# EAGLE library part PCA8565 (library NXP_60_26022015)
Real time clock/calendar The PCA8565 is a CMOS real time clock and calendar optimized for low power consumption. A programmable clock output, interrupt output and voltage-low detector are also provided. All address and data are transferred serially via a two-line bidirectional I2C-bus. Maximum bus speed is 400 kbit/s. The built-in word address register is incremented automatically after each written or read data byte. AEC-Q100 compliant (PCA8565TS) for automotive applications. AAL Eindhoven MK
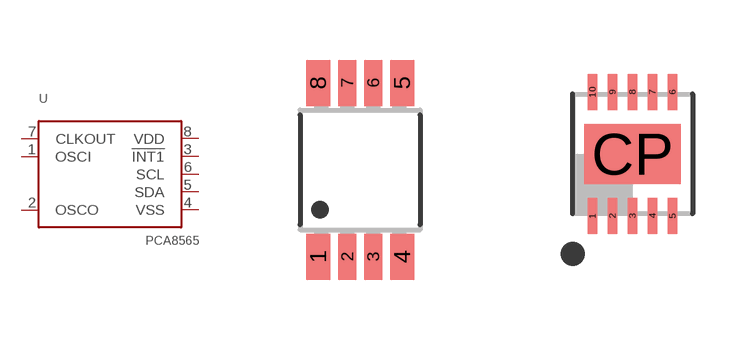
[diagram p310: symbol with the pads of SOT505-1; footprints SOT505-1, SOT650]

Designator prefix U

## PCA8565TS  [SOT505-1]
1  OSCI  pas
2  OSCO  pas
3  !INT1!  out
4  VSS  pwr
5  SDA
6  SCL  in
7  CLKOUT  pwr
8  VDD  pwr

## PCA8565BS  [SOT650]
1  OSCI  pas
2  OSCO  pas
4  !INT1!  out
5  VSS  pwr
6  SDA
7  SCL  in
8  CLKOUT  pwr
9  VDD  pwr

## Footprint SOT505-1 (pad centres in mm)
SOT505-1 TSSOP8: plastic thin shrink small outline package; 8 leads; body width 3 mm JEDEC: -- IEC: --
smd 0.6 x 1.15: 1 -1.05,-2.175; 4 1.05,-2.175; 5 1.05,2.175; 8 -1.05,2.175
smd 0.45 x 1.15: 2 -0.325,-2.175; 3 0.325,-2.175; 6 0.325,2.175; 7 -0.325,2.175

## Footprint SOT650 (pad centres in mm)
SOT650 HVSON10: plastic thermal enhanced very thin small outline package; no leads; 10 terminals; body 3 x 3 x 0.85 mm JEDEC: MO-229 IEC: -- JEITA:--
smd 0.24 x 0.9: 1 -1,-1.55; 2 -0.5,-1.55; 3 0,-1.55; 4 0.5,-1.55; 5 1,-1.55; 6 1,1.55; 7 0.5,1.55; 8 0,1.55; 9 -0.5,1.55; 10 -1,1.55
smd 2.4 x 1.5: CP 0,0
